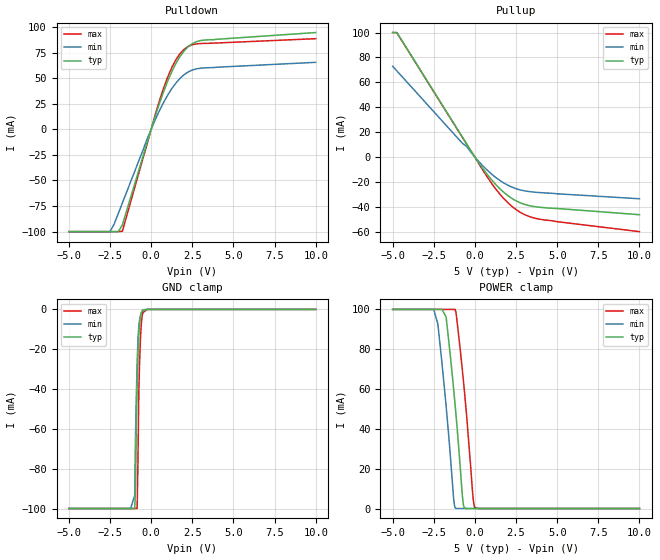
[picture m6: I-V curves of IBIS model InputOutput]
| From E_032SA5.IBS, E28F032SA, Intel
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|***********************Input Output Model***********************
[Model]   InputOutput
Model_type   I/O
|   for DQ[15:0]
Vinl = 0.8V
Vinh = 2.0V
| Variable   typ   min   max
C_comp   9.61p   NA   11.6p
[Voltage Range]   5.0V   4.5V   5.5V
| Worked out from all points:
|   slope of the pulldown table from 0 to 0.75 V, typ, clamps not added: 20.6 ohm
|   slope of the pullup table from 0 to 0.75 V, typ, clamps not added: 53.7 ohm
|   GND clamp passes 1 mA (typ) near -0.54 V on its own axis
|   POWER clamp passes 1 mA (typ) near -0.67 V on its own axis
[Pulldown]
| [Pullup] and [Pulldown] IV curves include only the current through
| the channels of output driver transistors when outputs are enabled
| with OE# = VIL.  Although the output driver transistors have np and
| pn diodes inherently created by CMOS IC fabrication between the
| drain and bulk of n-channel and p-channel CMOS transistors,
| the current through these junction diodes is not included in
| [Pullup] or [Pulldown].  Instead that drain/bulk diode current is
| included in the [POWER_clamp] or [GND_clamp] sections, which are
| not dependent on the state of OE# or output data value.
|Voltage  I(typ)   I(min)   I(max)
-5V       -100mA     -100mA     -100mA
-2.5V     -100mA     -100mA     -100mA
-2V       -100mA     -82.4mA    -100mA
-1.75V    -93.52mA   -72.08mA   -99.6mA
-250mV    -13.38mA   -9.701mA   -14.76mA
250mV     12.96mA    9.398mA    14.42mA
750mV     36.49mA    26.01mA    39.96mA
1.5V      64.22mA    45.1mA     67.86mA
2V        76.48mA    53.32mA    78.14mA
2.5V      83.64mA    57.89mA    82.59mA
3V        86.64mA    59.65mA    83.77mA
10V       94.5mA     65.4mA     88.5mA
[GND_clamp]
| [POWER_clamp] and [GND_clamp] IV curves describe ESD protection
| circuits PLUS some np and pn diodes which exist between the
| drain and bulk of n-channel and p-channel CMOS transistors.
| These drain/bulk diodes are inherent in CMOS IC fabrication,
| and are visible on the node of the I/O pin at all times.
| Even the drain/bulk diodes of output driver [Pullup] and [Powerdown]
| transistors are included in [POWER_clamp] or [GND_clamp], because
| these diodes contribute to I/O pin current even when the
| chip outputs are tristated by OE# = VIH.
| For example, when V forced on the I/O pin is large, we are
| forward biasing the pn diode at the drain/bulk interface in the
| p-channel pullup transistor.  Similarly, when V forced on the
| I/O pin is sufficiently negative with respect to the substrate
| ground, we are forward biasing the np diode at the drain/bulk
| interface in the n-channel pulldown transistor.  The effects
| of these diodes are included in [POWER_clamp] or [GND_clamp].
|Voltage  I(typ)   I(min)   I(max)
-5V       -99.85mA   -99.86mA   -99.85mA
-1.25V    -99.85mA   -99.86mA   -99.85mA
-1V       -99.85mA   -93.36mA   -99.85mA
-950mV    -90.34mA   -63.24mA   -99.85mA
-900mV    -57.16mA   -42.82mA   -99.85mA
-850mV    -38.91mA   -26.66mA   -99.85mA
-800mV    -23.28mA   -14.71mA   -74.74mA
-750mV    -12.68mA   -8.348mA   -41.38mA
-700mV    -6.759mA   -5.06mA    -26.01mA
-600mV    -2.156mA   -1.643mA   -7.325mA
-500mV    -423.7uA   -221.5uA   -1.566mA
10V       0A         0A         0A
[Pullup]
| (Voltages for [Pullup] and [POWER_clamp] are specified with
| negative respect to Vcc.  Reference the IBIS documentation
| for more information regarding Vtable = Vcc - Voutput.
| This method keeps -Vds constant for the values in all three
| columns across a line of the table.
| [Pullup] and [Pulldown] IV curves include only the current through
| the channels of output driver transistors when outputs are enabled
| with OE# = VIL.  Although the output driver transistors have np and
| pn diodes inherently created by CMOS IC fabrication between the
| drain and bulk of n-channel and p-channel CMOS transistors,
| the current through these junction diodes is not included in
| [Pullup] or [Pulldown].  Instead that drain/bulk diode current is
| included in the [POWER_clamp] or [GND_clamp] sections, which are
| not dependent on the state of OE# or output data value.
|Voltage  I(typ)   I(min)   I(max)
-5V       100mA      72.96mA    100mA
-4.75V    100mA      69.31mA    99.93mA
-750mV    15.8mA     10.91mA    15.53mA
-500mV    10.57mA    8.552mA    10.25mA
250mV     -4.915mA   -3.791mA   -5.55mA
750mV     -13.97mA   -10.54mA   -16.02mA
1.25V     -21.8mA    -16.24mA   -25.38mA
2V        -30.94mA   -22.62mA   -36.66mA
2.75V     -36.71mA   -26.38mA   -44.34mA
3.25V     -38.84mA   -27.64mA   -47.51mA
3.75V     -40.02mA   -28.34mA   -49.44mA
10V       -46.3mA    -33.5mA    -59.9mA
[POWER_clamp]
| (Voltages for [Pullup] and [POWER_clamp] are specified with
| negative respect to Vcc.  Reference the IBIS documentation
| for more information regarding Vtable = Vcc - Voutput.
| This method keeps -Vds constant for the values in all three
| columns across a line of the table.
| [POWER_clamp] and [GND_clamp] IV curves describe ESD protection
| circuits PLUS some np and pn diodes which exist between the
| drain and bulk of n-channel and p-channel CMOS transistors.
| These drain/bulk diodes are inherent in CMOS IC fabrication,
| and are visible on the node of the I/O pin at all times.
| Even the drain/bulk diodes of output driver [Pullup] and [Powerdown]
| transistors are included in [POWER_clamp] or [GND_clamp], because
| these diodes contribute to I/O pin current even when the
| chip outputs are tristated by OE# = VIH.
| For example, when V forced on the I/O pin is large, we are
| forward biasing the pn diode at the drain/bulk interface in the
| p-channel pullup transistor.  Similarly, when V forced on the
| I/O pin is sufficiently negative with respect to the substrate
| ground, we are forward biasing the np diode at the drain/bulk
| interface in the n-channel pulldown transistor.  The effects
| of these diodes are included in [POWER_clamp] or [GND_clamp].
|Voltage  I(typ)   I(min)   I(max)
-5V       100mA      100mA      100mA
-2.5V     100mA      100mA      100mA
-2.25V    100mA      92.59mA    100mA
-1.75V    96.25mA    51.53mA    100mA
-1.3V     60.58mA    5.804mA    100mA
-1.2V     51.74mA    365.3uA    100mA
-1.1V     42.39mA    0A         95.1mA
-700mV    1.826mA    0A         64.4mA
-500mV    1.279uA    0A         46.44mA
-100mV    0A         0A         4.387mA
0V        0A         0A         398.5uA
10V       0A         0A         0A
[Ramp]
| The DQ Ramp information is not provided at this time for the
| device but will be available in the future.  The table below
| is for the compatibility with some IBIS parsers.
| Variable   typ   min   max
 dV/dt_r   0V/0ns   0V/0ns   0V/0ns
 dV/dt_f   0V/0ns   0V/0ns   0V/0ns
